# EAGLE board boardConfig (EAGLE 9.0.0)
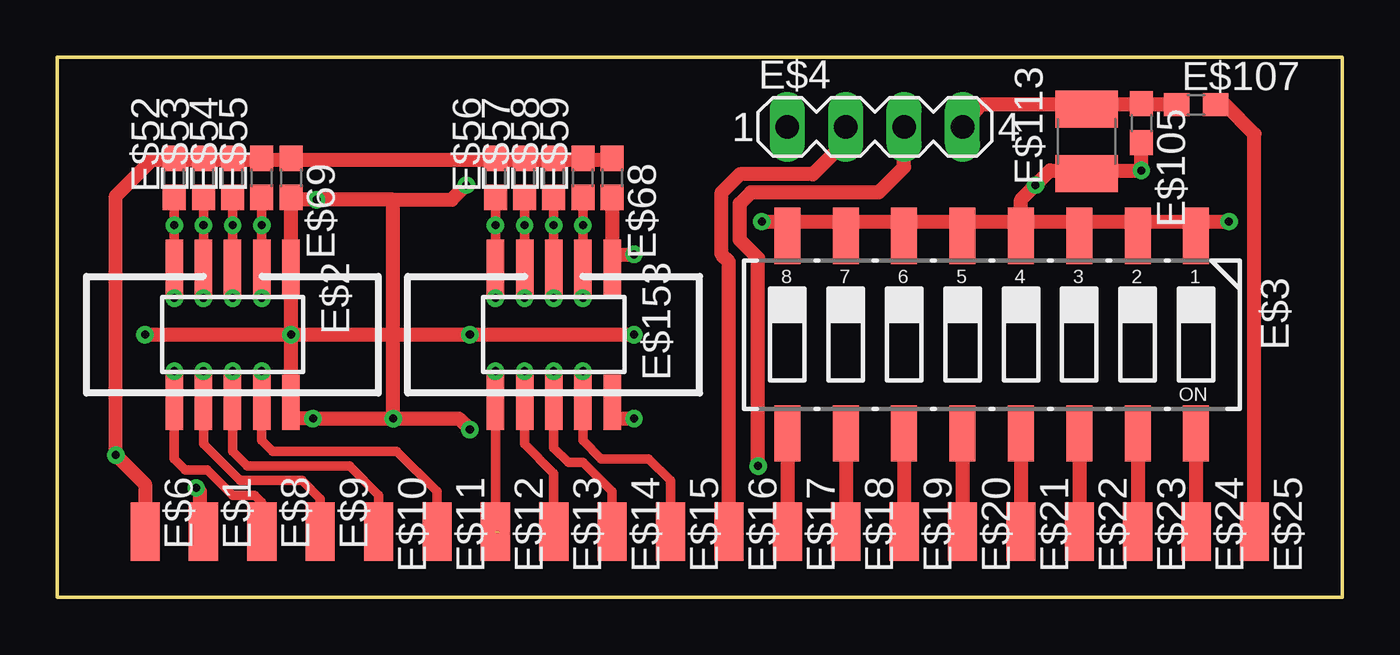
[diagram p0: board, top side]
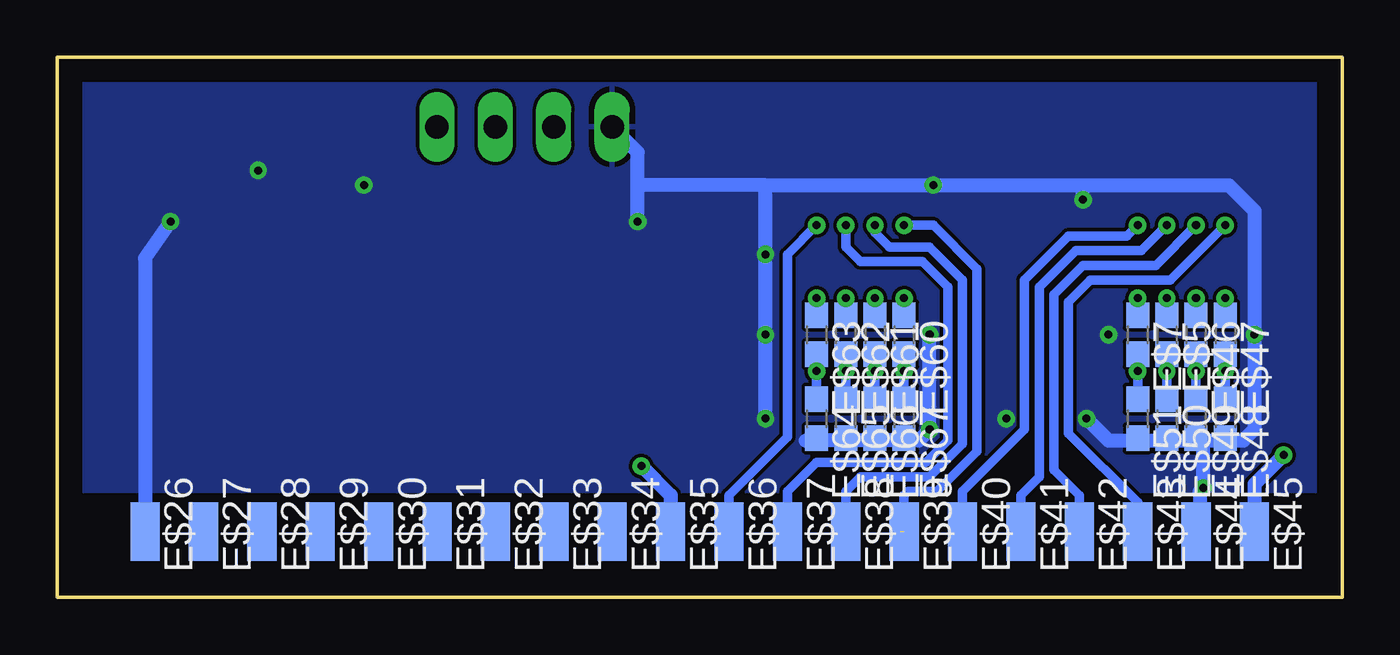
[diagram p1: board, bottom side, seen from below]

Size 55.88 x 23.49 mm. Coordinates in mm from the lower left corner, seen from the top.
Outline: 0,0 0,23.49 55.88,23.49 55.88,0 0,0
Copper layers (1+16): Top 0.035mm / dielectric 1.5mm / Bottom 0.035mm
Design rules "default *": minimum track width 6mil, minimum drill 0.35mm, track to track 6mil, track to pad 6mil, pad to pad 6mil, via to via 6mil, smd to smd 6mil, copper to edge 40mil, drill to drill 6mil, minimum pad ring 10mil, minimum via ring 8mil, stop-mask expansion 4mil, vias tented up to drill 0mil, thermal gap 10mil

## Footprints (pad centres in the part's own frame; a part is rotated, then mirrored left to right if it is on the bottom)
SMD1,27-2,54 = smd 1.27 x 2.54: 1 0,0
1365-10 = smd 0.76 x 2.4: 1 -2.54,-2.95; 2 -2.54,2.95; 3 -1.27,-2.95; 4 -1.27,2.95; 5 0,-2.95; 6 0,2.95; 7 1.27,-2.95; 8 1.27,2.95; 9 2.54,-2.95; 10 2.54,2.95
CTS-219-08 = smd 1.13 x 2.44: 1 -8.89,-4.3; 2 -6.35,-4.3; 3 -3.81,-4.3; 4 -1.27,-4.3; 5 1.27,-4.3; 6 3.81,-4.3; 7 6.35,-4.3; 8 8.89,-4.3; 9 8.89,4.3; 10 6.35,4.3; 11 3.81,4.3; 12 1.27,4.3; 13 -1.27,4.3; 14 -3.81,4.3; 15 -6.35,4.3; 16 -8.89,4.3
MA04-1 = drill 1.016 long: 1 -3.81,0; 2 -1.27,0; 3 1.27,0; 4 3.81,0
C0603 = smd 1.1 x 1: 1 -0.85,0; 2 0.85,0
C1210 = smd 1.6 x 2.7: 1 -1.4,0; 2 1.4,0

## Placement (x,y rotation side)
E$1  [SMD1,27-2,54]  6.35,2.86 180 top
E$2  Connector 10 pin  [1365-10]  7.62,11.43 180 top
E$3  [CTS-219-08]  40.64,11.43 180 top
E$4  [MA04-1]  35.56,20.48 0 top
E$5  1.5K  [C0603]  7.62,11.43 270 bottom
E$6  [SMD1,27-2,54]  3.81,2.86 180 top
E$7  1.5K  [C0603]  8.89,11.43 270 bottom
E$8  [SMD1,27-2,54]  8.89,2.86 180 top
E$9  [SMD1,27-2,54]  11.43,2.86 180 top
E$10  [SMD1,27-2,54]  13.97,2.86 180 top
E$11  [SMD1,27-2,54]  16.51,2.86 180 top
E$12  [SMD1,27-2,54]  19.05,2.86 180 top
E$13  [SMD1,27-2,54]  21.59,2.86 180 top
E$14  [SMD1,27-2,54]  24.13,2.86 180 top
E$15  [SMD1,27-2,54]  26.67,2.86 180 top
E$16  [SMD1,27-2,54]  29.21,2.86 180 top
E$17  [SMD1,27-2,54]  31.75,2.86 180 top
E$18  [SMD1,27-2,54]  34.29,2.86 180 top
E$19  [SMD1,27-2,54]  36.83,2.86 180 top
E$20  [SMD1,27-2,54]  39.37,2.86 180 top
E$21  [SMD1,27-2,54]  41.91,2.86 180 top
E$22  [SMD1,27-2,54]  44.45,2.86 180 top
E$23  [SMD1,27-2,54]  46.99,2.86 180 top
E$24  [SMD1,27-2,54]  49.53,2.86 180 top
E$25  [SMD1,27-2,54]  52.07,2.86 180 top
E$26  [SMD1,27-2,54]  52.07,2.86 180 bottom
E$27  [SMD1,27-2,54]  49.53,2.86 180 bottom
E$28  [SMD1,27-2,54]  46.99,2.86 180 bottom
E$29  [SMD1,27-2,54]  44.45,2.86 180 bottom
E$30  [SMD1,27-2,54]  41.91,2.86 180 bottom
E$31  [SMD1,27-2,54]  39.37,2.86 180 bottom
E$32  [SMD1,27-2,54]  36.83,2.86 180 bottom
E$33  [SMD1,27-2,54]  34.29,2.86 180 bottom
E$34  [SMD1,27-2,54]  31.75,2.86 180 bottom
E$35  [SMD1,27-2,54]  29.21,2.86 180 bottom
E$36  [SMD1,27-2,54]  26.67,2.86 180 bottom
E$37  [SMD1,27-2,54]  24.13,2.86 180 bottom
E$38  [SMD1,27-2,54]  21.59,2.86 180 bottom
E$39  [SMD1,27-2,54]  19.05,2.86 180 bottom
E$40  [SMD1,27-2,54]  16.51,2.86 180 bottom
E$41  [SMD1,27-2,54]  13.97,2.86 180 bottom
E$42  [SMD1,27-2,54]  11.43,2.86 180 bottom
E$43  [SMD1,27-2,54]  8.89,2.86 180 bottom
E$44  [SMD1,27-2,54]  6.35,2.86 180 bottom
E$45  [SMD1,27-2,54]  3.81,2.86 180 bottom
E$46  1.5K  [C0603]  6.35,11.43 270 bottom
E$47  1.5K  [C0603]  5.08,11.43 270 bottom
E$48  2.2K  [C0603]  5.08,7.78 270 bottom
E$49  2.2K  [C0603]  6.35,7.78 270 bottom
E$50  2.2K  [C0603]  7.62,7.78 270 bottom
E$51  2.2K  [C0603]  8.89,7.78 270 bottom
E$52  6.8K  [C0603]  5.08,18.26 90 top  (not fitted)
E$53  6.8K  [C0603]  6.35,18.26 90 top  (not fitted)
E$54  6.8K  [C0603]  7.62,18.26 90 top  (not fitted)
E$55  6.8K  [C0603]  8.89,18.26 90 top  (not fitted)
E$56  6.8K  [C0603]  19.05,18.26 90 top  (not fitted)
E$57  6.8K  [C0603]  20.32,18.26 90 top  (not fitted)
E$58  6.8K  [C0603]  21.59,18.26 90 top  (not fitted)
E$59  6.8K  [C0603]  22.86,18.26 90 top  (not fitted)
E$60  1.5K  [C0603]  19.05,11.43 270 bottom
E$61  1.5K  [C0603]  20.32,11.43 270 bottom
E$62  1.5K  [C0603]  21.59,11.43 270 bottom
E$63  1.5K  [C0603]  22.86,11.43 270 bottom
E$64  1K  [C0603]  22.86,7.78 270 bottom
E$65  1K  [C0603]  21.59,7.78 270 bottom
E$66  1K  [C0603]  20.32,7.78 270 bottom
E$67  1K  [C0603]  19.05,7.78 270 bottom
E$68  100nF  [C0603]  24.13,18.26 270 top  (not fitted)
E$69  100nF  [C0603]  10.16,18.26 270 top
E$105  100nF  [C0603]  47.15,20.64 270 top
E$107  Ferrit/470R  [C0603]  49.53,21.43 0 top
E$113  100uF/16V  [C1210]  44.77,19.84 90 top
E$153  Connector 10 pin  [1365-10]  21.59,11.43 180 top

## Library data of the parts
E$1 E$6 E$8-E$45 = wirepad
E$2 E$153 = con-leotronics
E$3 = switch-dil
E$4 = con-lstb
E$5 E$7 E$46-E$69 E$105 E$107 E$113 = rcl

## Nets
3.3V: E$6.1 E$45.1
5V_2: E$4.4
DIP0: E$24.1
DIP1: E$23.1
DIP2: E$22.1
DIP4: E$20.1
DIP6: E$18.1
DIP7: E$17.1
FAN1: E$4.2 E$16.1
FAN2: E$4.3 E$35.1
GND: E$4.1
S0_1N: E$40.1
S0_1P: E$11.1
S0_2N: E$36.1
S0_2P: E$15.1
S1_1N: E$41.1
S1_1P: E$10.1
S1_2N: E$37.1
S1_2P: E$14.1
S2_1N: E$42.1
S2_1P: E$9.1
S2_2N: E$38.1
S2_2P: E$13.1
S3_1P: E$8.1
S3_2N: E$39.1
S3_2P: E$12.1

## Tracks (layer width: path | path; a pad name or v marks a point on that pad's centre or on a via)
3.3V  (via drill 0.35)
  Top 0.61: E$45.1 3.81,4.92 v2.54,6.19 2.54,17.46 4.13,19.05 24.29,19.05
  Bottom 0.61: v2.54,6.19 3.81,4.92 E$45.1
5V_2
  Top 0.61: 48.58,21.43 40.16,21.43 E$4.4
+5V
  Top 0.61: 50.8,21.43 52.07,20.16 52.07,3.02
DIP0
  Top 0.61: 49.53,6.99 E$24.1
DIP1
  Top 0.61: 46.99,6.99 E$23.1
DIP2
  Top 0.61: 44.45,6.99 E$22.1
DIP3
  Top 0.61: 41.91,7.14 41.91,2.86
DIP4
  Top 0.61: 39.37,6.99 E$20.1
DIP5
  Top 0.61: 36.83,6.83 36.83,2.7
DIP6
  Top 0.61: 34.29,6.99 E$18.1
DIP7
  Top 0.61: 31.75,6.99 E$17.1
FAN1
  Top 0.61: E$16.1 29.21,14.6 28.89,14.92 28.89,17.62 29.69,18.41 32.86,18.41 34.29,19.84 E$4.2
FAN2  (via drill 0.35)
  Top 0.61: v30.48,5.71 30.48,14.76 29.69,15.56 29.69,17.14 30.16,17.62 35.72,17.62 36.83,18.73 E$4.3
  Bottom 0.61: v30.48,5.71 29.21,4.44 E$35.1
GND  (via drill 0.35)
  Top 0.61: v30.64,16.35 41.91,16.35 | 41.91,16.35 v50.96,16.35 | 41.91,16.35 41.91,17.3 v42.55,17.94 43.18,18.57 v47.15,18.57 47.15,19.69 | 24.13,7.78 v25.08,7.78 | v25.08,14.92 24.13,14.92 24.13,17.3 | v6.03,4.76 6.19,4.6 6.19,2.7 | v25.08,11.43 v17.94,11.43 14.61,11.43 | v10.16,11.43 10.16,7.78 v11.11,7.78 v14.61,7.78 | v10.16,11.43 10.16,17.3 v11.27,17.3 14.61,17.3 | v3.81,11.43 v10.16,11.43 | v10.16,11.43 14.61,11.43 | v14.61,7.78 17.46,7.78 v17.94,7.3 | v14.61,7.78 14.61,11.43 | 14.61,11.43 14.61,17.3 | 14.61,17.3 17.14,17.3 v17.78,17.94
  Bottom 0.61: v50.96,16.35 52.07,14.76 52.07,3.02 | 25.08,17.94 v17.78,17.94 11.27,17.94 | 11.27,17.94 4.92,17.94 3.81,16.83 v3.81,11.43 3.81,7.3 4.29,6.83 6.03,6.83 | v30.64,16.35 30.64,17.94 | 30.64,17.94 30.64,19.37 E$4.1 | v25.08,7.78 v25.08,11.43 v25.08,14.92 25.08,17.94 | 25.08,17.94 30.64,17.94 | 6.19,2.7 6.19,4.6 v6.03,4.76 6.03,6.83 | 6.03,6.83 10.16,6.83 v11.11,7.78 | 17.94,7.46 v17.94,11.43 | v17.94,7.3 18.42,6.83 23.34,6.83 | v11.27,17.3 11.27,17.94
  pour Bottom: 0,4.6 55.88,4.6 55.88,23.49 0,23.49
S0_1N  (via drill 0.35)
  Top 0.406: 8.89,17.46 v8.89,16.19 v8.89,13.02
  Bottom 0.406: v8.89,16.19 9.37,15.72 11.91,15.72 13.81,13.81 13.81,7.3 16.51,4.6 16.51,3.18 | v8.89,13.02 8.89,12.22
  Bottom 0.61: 16.51,3.18 E$40.1
S0_1P  (via drill 0.35)
  Top 0.406: E$11.1 16.51,4.6 14.76,6.35 9.37,6.35 8.89,6.83 v8.89,9.84
  Bottom 0.406: 8.89,8.89 v8.89,9.84 8.89,10.48
S0_2N  (via drill 0.35)
  Top 0.406: 22.86,17.46 v22.86,16.19 v22.86,13.02
  Bottom 0.406: v22.86,13.02 22.86,12.38 | 26.67,3.97 E$36.1 26.67,4.44 24.13,6.99 24.13,14.92 v22.86,16.19
S0_2P  (via drill 0.35)
  Top 0.406: E$15.1 26.67,5.08 25.72,6.03 23.65,6.03 22.86,6.83 22.86,7.3 22.86,8.25 v22.86,9.84
  Bottom 0.406: 22.86,10.64 v22.86,9.84 22.86,8.89
S1_1N  (via drill 0.35)
  Top 0.406: 7.62,17.46 v7.62,16.19 v7.62,13.02
  Bottom 0.406: v7.62,16.19 8.73,15.08 11.59,15.08 13.18,13.49 13.18,5.24 13.97,4.44 13.97,3.33 | v7.62,13.02 7.62,12.22
  Bottom 0.61: 13.97,3.33 E$41.1
S1_1P  (via drill 0.35)
  Top 0.406: E$10.1 13.97,4.44 12.7,5.71 8.25,5.71 7.62,6.35 v7.62,9.84
  Bottom 0.406: 7.62,8.73 v7.62,9.84 7.62,10.48
S1_2N  (via drill 0.35)
  Top 0.406: 21.59,17.46 v21.59,16.19 v21.59,13.02
  Bottom 0.406: v21.59,13.02 21.59,12.38 | E$37.1 24.13,4.6 22.86,5.87 18.1,5.87 17.14,6.83 17.14,13.49 18.26,14.6 20.96,14.6 21.59,15.24 v21.59,16.19
S1_2P  (via drill 0.35)
  Top 0.406: v21.59,9.84 21.59,6.51 22.22,5.87 22.86,5.87 24.13,4.6 E$14.1 24.13,3.97
  Bottom 0.406: 21.59,10.64 v21.59,9.84 21.59,8.89
S2_1N  (via drill 0.35)
  Top 0.406: 6.35,17.46 v6.35,16.19 v6.35,13.02
  Bottom 0.406: v6.35,13.02 6.35,12.22 | v6.35,16.19 8.1,14.45 11.27,14.45 12.54,13.18 12.54,5.56 11.43,4.44 11.43,3.02
  Bottom 0.61: 11.43,3.02 E$42.1
S2_1P  (via drill 0.35)
  Top 0.406: E$9.1 11.43,4.29 10.64,5.08 7.94,5.08 6.35,6.67 v6.35,9.84
  Bottom 0.406: 6.35,8.89 v6.35,9.84 6.35,10.64
S2_2N  (via drill 0.35)
  Top 0.406: 20.32,17.46 v20.32,16.19 v20.32,13.02
  Bottom 0.406: v20.32,13.02 20.32,12.38 | E$38.1 21.59,4.6 20.96,5.24 17.94,5.24 16.51,6.67 16.51,13.81 17.94,15.24 19.68,15.24 20.32,15.88 v20.32,16.19
S2_2P  (via drill 0.35)
  Top 0.406: v20.32,9.84 20.32,6.67 21.59,5.4 E$13.1
  Bottom 0.406: 20.32,10.64 v20.32,9.84 20.32,8.89
S3_1N  (via drill 0.35)
  Top 0.406: 5.08,17.46 v5.08,16.19 v5.08,13.02
  Bottom 0.406: v5.08,16.19 7.46,13.81 10.95,13.81 11.91,12.86 11.91,7.14 8.89,4.13 | v5.08,13.02 5.08,12.22
S3_1P  (via drill 0.35)
  Top 0.406: E$8.1 8.89,4.13 8.57,4.44 7.62,4.44 6.51,5.56 5.56,5.56 5.08,6.03 v5.08,9.84
  Bottom 0.406: 5.08,8.73 v5.08,9.84 5.08,10.64
S3_2N  (via drill 0.35)  (1 unrouted)
  Top 0.406: 19.05,17.46 v19.05,16.19 v19.05,13.02
  Bottom 0.406: v19.05,13.02 19.05,12.38 | v19.05,16.19 17.78,16.19 15.87,14.29 15.87,6.35 17.62,4.6 18.89,4.6 19.05,4.44 E$39.1 | 19.21,2.86 19.21,3.18
S3_2P  (via drill 0.35)
  Top 0.406: E$12.1 v19.05,9.84
  Bottom 0.406: 19.05,10.64 v19.05,9.84 19.05,9.05

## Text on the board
Document: Link 1 | Link 2 | GND | 5V | Vers2 | 1 | 0 | bit7 | bit0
